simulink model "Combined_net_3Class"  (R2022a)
settings: Solver=FixedStepAuto  StartTime=0.0  StopTime=simtime  FixedStep=1  RelTol=1e-3
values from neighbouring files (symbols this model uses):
  simtime = length(SOC_CC{1, 1})    [Data_preparation.m]    (also in SimulationCycle.m = cell2mat(simtime_og(i)))
  SOH_predict = double(ans.SOHout(simtime))    [SimulationCycle.m]
undefined symbols (not defined in the file or in its folder): dSOC_mu_CC, dSOC_sig_CC, dv_mu_CC, dv_sig_CC, SOC_mu_CC, SOC_sig_CC, SOE_mu_CC, SOE_sig_CC
libraries: neural x121, deeplib x1
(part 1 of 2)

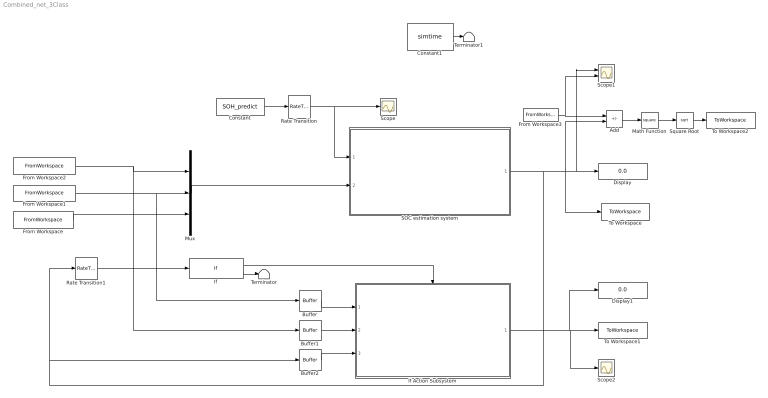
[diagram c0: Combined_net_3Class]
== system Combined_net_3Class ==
  Add : Sum  Inputs=+-
  Buffer : Buffer  N=120  OutputFrames=off
  Buffer1 : Buffer  N=120  OutputFrames=off
  Buffer2 : Buffer  N=120  OutputFrames=off
  Constant : Constant  Value=SOH_predict
  Constant1 : Constant  Value=simtime
  Display : Display
  Display1 : Display
  From Workspace : FromWorkspace  VariableName=Temperature
  From Workspace1 : FromWorkspace  VariableName=Voltage  SampleTime=1
  From Workspace2 : FromWorkspace  VariableName=Current  SampleTime=1
  From Workspace3 : FromWorkspace  VariableName=SOC_GT
  If : If  IfExpression=u1 < 0.6
  If Action Subsystem : Subsystem  TreatAsAtomicUnit=on
  Math Function : Math  Operator=square
  Mux : Mux  Inputs=3
  Rate Transition : RateTransition  OutPortSampleTime=1
  Rate Transition1 : RateTransition  OutPortSampleTime=1
  SOC estimation system : Subsystem
  Scope : Scope
  Scope1 : Scope  NumInputPorts=2
  Scope2 : Scope
  Square Root : Sqrt
  Terminator : Terminator
  Terminator1 : Terminator
  To Workspace : ToWorkspace  VariableName=SOCout  SampleTime=-1
  To Workspace1 : ToWorkspace  VariableName=SOHout  SampleTime=-1
  To Workspace2 : ToWorkspace  VariableName=SOC_abserror  SampleTime=-1
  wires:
  From Workspace/1 -> Mux/3
  Mux/1 -> SOC estimation system/2(Input data)
  If/1 -> If Action Subsystem/Action
  If/2 -> Terminator/1
  Rate Transition1/1 -> If/1
  Buffer2/1 -> If Action Subsystem/3(SOC)
  Buffer1/1 -> If Action Subsystem/2(I)
  From Workspace1/1 -> Buffer/1, Mux/2
  Buffer/1 -> If Action Subsystem/1(V)
  SOC estimation system/1(SOC) -> Scope1/1, Display/1, Add/2, To Workspace/1, Buffer2/1, Rate Transition1/1
  From Workspace2/1 -> Mux/1, Buffer1/1
  If Action Subsystem/1(SOH) -> Display1/1, Scope2/1, To Workspace1/1
  Add/1 -> Math Function/1
  Math Function/1 -> Square Root/1
  Square Root/1 -> To Workspace2/1
  Constant1/1 -> Terminator1/1
  Rate Transition/1 -> SOC estimation system/1(SOH), Scope/1
  From Workspace3/1 -> Add/1, Scope1/2
  Constant/1 -> Rate Transition/1

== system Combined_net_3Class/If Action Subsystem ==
  V : Inport
  I : Inport  Port=2
  SOC : Inport  Port=3
  Action Port : ActionPort  ActionPortLabel=if(u1 < 0.7)
  SOH estimation system : Subsystem
  SOH : Outport
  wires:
  V/1 -> SOH estimation system/1(V)
  I/1 -> SOH estimation system/2(I)
  SOC/1 -> SOH estimation system/3(SOC)
  SOH estimation system/1(Input1) -> SOH/1

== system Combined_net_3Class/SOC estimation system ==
  SOH : Inport
  Input data : Inport  Port=2
  Class1 : Subsystem  TreatAsAtomicUnit=on
  Class2 : Subsystem  TreatAsAtomicUnit=on
  Class3 : Subsystem  TreatAsAtomicUnit=on
  If : If  IfExpression=u1 > 0.93  ElseIfExpressions=u1 <= 0.93 & u1>0.9
  Merge : Merge  Inputs=3
  SOC : Outport
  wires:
  Class2/1(Output) -> Merge/2
  If/1 -> Class1/Action
  Merge/1 -> SOC/1
  Class3/1(Output) -> Merge/3
  Class1/1(Output) -> Merge/1
  SOH/1 -> If/1
  Input data/1 -> Class3/1(Input), Class2/1(Input), Class1/1(Input)
  If/2 -> Class2/Action
  If/3 -> Class3/Action

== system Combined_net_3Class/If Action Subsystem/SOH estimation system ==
  V : Inport
  I : Inport  Port=2
  SOC : Inport  Port=3
  Subsystem1 : Subsystem
  Subsystem2 : Subsystem
  Input1 : Outport
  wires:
  Subsystem1/4(SOE) -> Subsystem2/4(SOE)
  Subsystem1/1(dSOC) -> Subsystem2/1(dSOC)
  Subsystem1/2(dv) -> Subsystem2/2(dv)
  Subsystem1/3(SOC) -> Subsystem2/3(SOC)
  Subsystem2/1(Input1) -> Input1/1
  V/1 -> Subsystem1/1(V_03)
  I/1 -> Subsystem1/2(I_03)
  SOC/1 -> Subsystem1/3(SOC_03)

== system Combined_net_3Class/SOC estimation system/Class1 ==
  Input : Inport
  Action Port : ActionPort  ActionPortLabel=if(u1 > 0.93)
  NARX Neural Network : Subsystem  mask{pi_input_1_delayed_1=[0.507169576059850246707583210081793367862701416015625;-0.464363636363636533843646247987635433673858642578125;-0.84734133790737542479831745367846451699733734130859375], ai_layer_2_delayed_1=-0.99999444038800466838523561818874441087245941162109375}
      mask prompts: pi_input_1_delayed_1 "Preprocessed initial input 1 state at timestep 0."; ai_layer_2_delayed_1 "Initial layer 2 state at timestep 0."
      mask help: NARX Neural Network
  Scope : Scope
  Output : Outport
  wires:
  Input/1 -> NARX Neural Network/1(x)
  NARX Neural Network/1(y) -> Scope/1, Output/1

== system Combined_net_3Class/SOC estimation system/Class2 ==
  Input : Inport
  Action Port : ActionPort  ActionPortLabel=elseif(u1 <= 0.93 & u1>0.9)
  Best class2 NARX Neural Network : Subsystem  mask{pi_input_1_delayed_1=[0.5045468798996550763291679686517454683780670166015625;-0.611404153034653230491812792024575173854827880859375;-1.2613636363636360204765196613152511417865753173828125], ai_layer_2_delayed_1=-0.999993347694183132290390858543105423450469970703125}
      mask prompts: pi_input_1_delayed_1 "Preprocessed initial input 1 state at timestep 0."; ai_layer_2_delayed_1 "Initial layer 2 state at timestep 0."
      mask help: NARX Neural Network
  Scope : Scope
  Output : Outport
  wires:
  Input/1 -> Best class2 NARX Neural Network/1(x)
  Best class2 NARX Neural Network/1(y) -> Scope/1, Output/1

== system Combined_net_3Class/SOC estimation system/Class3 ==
  Input : Inport
  Action Port : ActionPort  ActionPortLabel=else
  New Class 3 NARX Neural Network : Subsystem  mask{pi_input_1_delayed_1=[0.515744420666462755065140299848280847072601318359375;-0.590428999869605064532152027823030948638916015625;-0.633404864091559272054610119084827601909637451171875], ai_layer_2_delayed_1=-0.9999915611182650376775882250512950122356414794921875}
      mask prompts: pi_input_1_delayed_1 "Preprocessed initial input 1 state at timestep 0."; ai_layer_2_delayed_1 "Initial layer 2 state at timestep 0."
      mask help: NARX Neural Network
  Scope : Scope
  Output : Outport
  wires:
  Input/1 -> New Class 3 NARX Neural Network/1(x)
  New Class 3 NARX Neural Network/1(y) -> Scope/1, Output/1

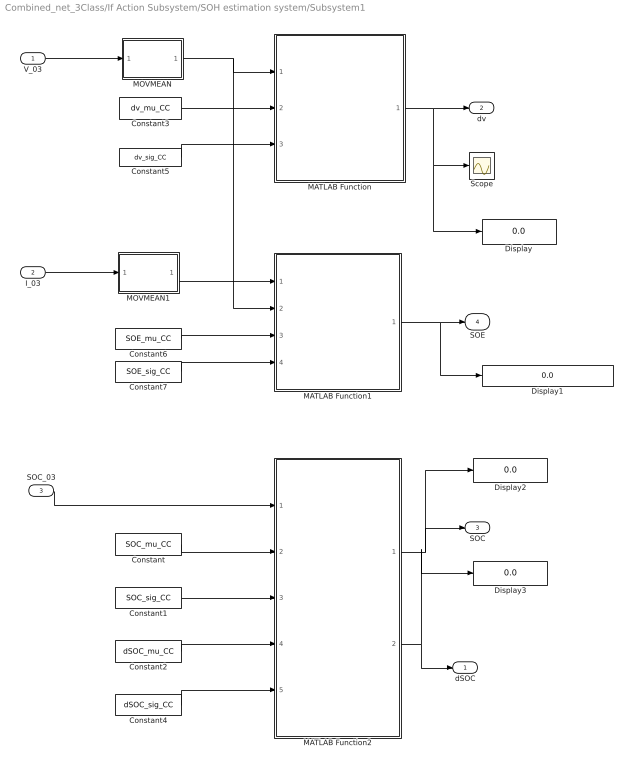
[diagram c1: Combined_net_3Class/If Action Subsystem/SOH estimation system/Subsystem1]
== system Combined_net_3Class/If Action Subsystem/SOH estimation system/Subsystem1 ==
  V_03 : Inport
  I_03 : Inport  Port=2
  SOC_03 : Inport  Port=3
  Constant : Constant  Value=SOC_mu_CC
  Constant1 : Constant  Value=SOC_sig_CC
  Constant2 : Constant  Value=dSOC_mu_CC
  Constant3 : Constant  Value=dv_mu_CC
  Constant4 : Constant  Value=dSOC_sig_CC
  Constant5 : Constant  Value=dv_sig_CC
  Constant6 : Constant  Value=SOE_mu_CC
  Constant7 : Constant  Value=SOE_sig_CC
  Display{,1..3} (4 alike) : Display
  MATLAB Function : MATLAB Function  TreatAsAtomicUnit=on
  MATLAB Function1 : MATLAB Function  TreatAsAtomicUnit=on
  MATLAB Function2 : MATLAB Function  TreatAsAtomicUnit=on
  MOVMEAN : MATLAB Function  TreatAsAtomicUnit=on
  MOVMEAN1 : MATLAB Function  TreatAsAtomicUnit=on
  Scope : Scope
  dSOC : Outport
  dv : Outport  Port=2
  SOC : Outport  Port=3
  SOE : Outport  Port=4
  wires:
  Constant4/1 -> MATLAB Function2/5(dSOC_sig_CC)
  Constant6/1 -> MATLAB Function1/3(SOE_mu_CC)
  Constant7/1 -> MATLAB Function1/4(SOE_sig_CC)
  Constant2/1 -> MATLAB Function2/4(dSOC_mu_CC)
  Constant5/1 -> MATLAB Function/3(dv_sig_CC)
  MATLAB Function2/2(dSOC) -> Display3/1, dSOC/1
  MATLAB Function/1(dV) -> Display/1, Scope/1, dv/1
  MATLAB Function2/1(SOC) -> Display2/1, SOC/1
  Constant3/1 -> MATLAB Function/2(dv_mu_CC)
  V_03/1 -> MOVMEAN/1(V)
  I_03/1 -> MOVMEAN1/1(I)
  Constant1/1 -> MATLAB Function2/3(SOC_sig_CC)
  Constant/1 -> MATLAB Function2/2(SOC_mu_CC)
  MATLAB Function1/1(SOE) -> Display1/1, SOE/1
  MOVMEAN/1(V_filt) -> MATLAB Function/1(V_03), MATLAB Function1/2(V_03)
  MOVMEAN1/1(I_filt) -> MATLAB Function1/1(I_03)
  SOC_03/1 -> MATLAB Function2/1(SOC_03)

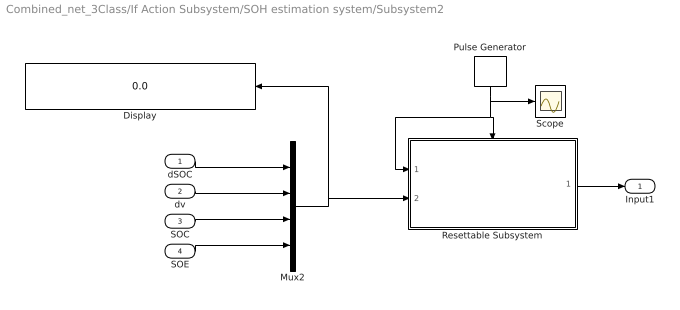
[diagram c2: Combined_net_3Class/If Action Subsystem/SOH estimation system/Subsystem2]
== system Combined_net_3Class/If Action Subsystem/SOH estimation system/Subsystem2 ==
  dSOC : Inport
  dv : Inport  Port=2
  SOC : Inport  Port=3
  SOE : Inport  Port=4
  Display : Display
  Mux2 : Mux
  Pulse Generator : DiscretePulseGenerator  PulseType=Time based  Period=120  PulseWidth=1/120*100  PhaseDelay=119
  Resettable Subsystem : Subsystem  TreatAsAtomicUnit=on
  Scope : Scope
  Input1 : Outport
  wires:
  Mux2/1 -> Display/1, Resettable Subsystem/2(Input1)
  dSOC/1 -> Mux2/1
  dv/1 -> Mux2/2
  SOC/1 -> Mux2/3
  SOE/1 -> Mux2/4
  Pulse Generator/1 -> Resettable Subsystem/1(Input), Resettable Subsystem/Reset, Scope/1
  Resettable Subsystem/1(Out1) -> Input1/1

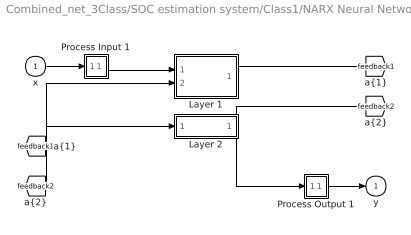
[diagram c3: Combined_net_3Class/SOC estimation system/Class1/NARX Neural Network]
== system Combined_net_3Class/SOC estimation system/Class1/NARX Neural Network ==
  x : Inport  PortDimensions=3  SampleTime=1
  Layer 1 : Subsystem
  Layer 2 : Subsystem
  Process Input 1 : Subsystem
  Process Output 1 : Subsystem
  y : Outport  InitialOutput=0
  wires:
  x/1 -> Process Input 1/1(x)
  Process Output 1/1(y) -> y/1
  Process Input 1/1(p) -> Layer 1/1("p{1}")
  Layer 1/1("a{1}") -> [feedback1]
  [feedback1] -> Layer 2/1("a{1} ")
  Layer 2/1("a{2}") -> [feedback2], Process Output 1/1(a)
  [feedback2] -> Layer 1/2("a{2} ")

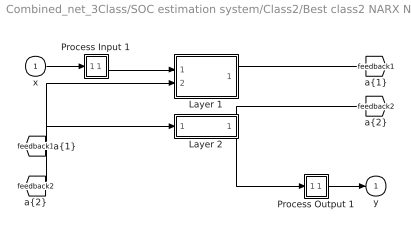
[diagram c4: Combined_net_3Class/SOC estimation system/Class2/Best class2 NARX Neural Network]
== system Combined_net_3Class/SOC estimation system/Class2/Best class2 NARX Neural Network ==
  x : Inport  PortDimensions=3  SampleTime=1
  Layer 1 : Subsystem
  Layer 2 : Subsystem
  Process Input 1 : Subsystem
  Process Output 1 : Subsystem
  y : Outport  InitialOutput=0
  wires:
  x/1 -> Process Input 1/1(x)
  Process Output 1/1(y) -> y/1
  Process Input 1/1(p) -> Layer 1/1("p{1}")
  Layer 1/1("a{1}") -> [feedback1]
  [feedback1] -> Layer 2/1("a{1} ")
  Layer 2/1("a{2}") -> [feedback2], Process Output 1/1(a)
  [feedback2] -> Layer 1/2("a{2} ")

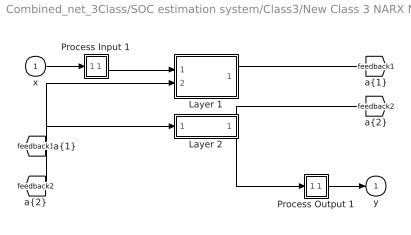
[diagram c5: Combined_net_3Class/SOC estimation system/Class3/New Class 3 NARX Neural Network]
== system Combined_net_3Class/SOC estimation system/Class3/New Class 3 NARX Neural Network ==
  x : Inport  PortDimensions=3  SampleTime=1
  Layer 1 : Subsystem
  Layer 2 : Subsystem
  Process Input 1 : Subsystem
  Process Output 1 : Subsystem
  y : Outport  InitialOutput=0
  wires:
  x/1 -> Process Input 1/1(x)
  Process Output 1/1(y) -> y/1
  Process Input 1/1(p) -> Layer 1/1("p{1}")
  Layer 1/1("a{1}") -> [feedback1]
  [feedback1] -> Layer 2/1("a{1} ")
  Layer 2/1("a{2}") -> [feedback2], Process Output 1/1(a)
  [feedback2] -> Layer 1/2("a{2} ")

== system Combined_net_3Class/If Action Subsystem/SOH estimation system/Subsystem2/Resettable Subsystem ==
  Input : Inport
  Input1 : Inport  Port=2
  Reset : ResetPort  DisableCoverage=on
  Triggered Subsystem : Subsystem  TreatAsAtomicUnit=on
  Out1 : Outport
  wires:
  Triggered Subsystem/1(Out1) -> Out1/1
  Input/1 -> Triggered Subsystem/Trigger
  Input1/1 -> Triggered Subsystem/1(u)

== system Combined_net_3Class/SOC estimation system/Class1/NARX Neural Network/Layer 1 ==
  "p{1}" : Inport  PortDimensions=3  SampleTime=1
  "a{2} " : Inport  Port=2  PortDimensions=1  SampleTime=1
  Delays 1 : Subsystem
  Delays 2 : Subsystem
  "IW{1,1}" : Subsystem
  "LW{1,2}" : Subsystem
  "b{1}" : Constant  Value=[2.272653460716699935773021934437565505504608154296875;1.38176429109038512166307555162347853183746337890625;-1.2278331254825765039839780001784674823284149169921875;-1.605402571388738319768663131981156766414642333984375;-0.32597678534726692856082763682934455573558807373046875;-0.63053100268787576343498813002952374517917633056640625;0.87053292866093390234283333484199829399585723876953125;0.155692044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
  netsum : Sum  Inputs=3  InputSameDT=on  SaturateOnIntegerOverflow=on
  tansig : neural/Transfer Functions/tansig
  "a{1}" : Outport  InitialOutput=[0;0;0;0;0;0;0;0;0;0;0;0;0;0;0;0;0;0;0]
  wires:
  "p{1}"/1 -> Delays 1/1("p{1}")
  Delays 1/1("pd{1,1}") -> "IW{1,1}"/1("pd{1,1}")
  "IW{1,1}"/1("iz{1,1}") -> netsum/1
  "a{2} "/1 -> Delays 2/1("p{1}")
  Delays 2/1("pd{1,2}") -> "LW{1,2}"/1("ad{1,2}")
  "LW{1,2}"/1("lz{1,2}") -> netsum/2
  "b{1}"/1 -> netsum/3
  netsum/1 -> tansig/1
  tansig/1 -> "a{1}"/1

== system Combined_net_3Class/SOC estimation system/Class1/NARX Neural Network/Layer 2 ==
  "a{1} " : Inport  PortDimensions=19  SampleTime=1
  Delays 1 : Subsystem
  "LW{2,1}" : Subsystem
  "b{2}" : Constant  Value=0.1358078901175280017721291869747801683843135833740234375
  netsum : Sum  Inputs=2  InputSameDT=on  SaturateOnIntegerOverflow=on
  purelin : neural/Transfer Functions/purelin
  "a{2}" : Outport  InitialOutput=0
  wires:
  "a{1} "/1 -> Delays 1/1("p{2}")
  Delays 1/1("pd{2,1}") -> "LW{2,1}"/1("ad{2,1}")
  "LW{2,1}"/1("lz{2,1}") -> netsum/1
  "b{2}"/1 -> netsum/2
  netsum/1 -> purelin/1
  purelin/1 -> "a{2}"/1

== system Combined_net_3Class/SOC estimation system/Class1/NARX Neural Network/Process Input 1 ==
  x : Inport  PortDimensions=3  SampleTime=1
  mapminmax : neural/Processing Functions/mapminmax  xmin=[-4.82500000000000017763568394003;2.50609999999999999431565811392;17.9379999999999988347099133534]  xmax=[1.5909999999999999698019337302;4.15610000000000034958702599397;34.2620000000000004547473508865]  ymin=-1  ymax=1
  p : Outport  PortDimensions=3  SampleTime=1
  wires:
  x/1 -> mapminmax/1
  mapminmax/1 -> p/1

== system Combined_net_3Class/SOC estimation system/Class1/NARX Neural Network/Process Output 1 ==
  a : Inport  PortDimensions=1  SampleTime=1
  mapminmax_reverse : neural/Processing Functions/mapminmax_reverse  xmin=-2.77982597386409656609138757455e-06  xmax=1.00000440635255594123975697585  ymin=-1  ymax=1
  y : Outport  PortDimensions=1  SampleTime=1
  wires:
  a/1 -> mapminmax_reverse/1
  mapminmax_reverse/1 -> y/1

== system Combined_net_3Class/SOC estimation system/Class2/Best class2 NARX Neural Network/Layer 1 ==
  "p{1}" : Inport  PortDimensions=3  SampleTime=1
  "a{2} " : Inport  Port=2  PortDimensions=1  SampleTime=1
  Delays 1 : Subsystem
  Delays 2 : Subsystem
  "IW{1,1}" : Subsystem
  "LW{1,2}" : Subsystem
  "b{1}" : Constant  Value=[2.32536033197951841344774948083795607089996337890625;1.6088426828114605893205180109362117946147918701171875;1.839289132479468680259060420212335884571075439453125;1.1409513281229022307883269604644738137722015380859375;-0.84272780046289941235926335139083676040172576904296875;0.8169616653562676855671043085749261081218719482421875;0.8137484932039795726410602583200670778751373291015625;-0.243541688874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
  netsum : Sum  Inputs=3  InputSameDT=on  SaturateOnIntegerOverflow=on
  tansig : neural/Transfer Functions/tansig
  "a{1}" : Outport  InitialOutput=[0;0;0;0;0;0;0;0;0;0;0;0;0;0;0;0;0;0]
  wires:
  "p{1}"/1 -> Delays 1/1("p{1}")
  Delays 1/1("pd{1,1}") -> "IW{1,1}"/1("pd{1,1}")
  "IW{1,1}"/1("iz{1,1}") -> netsum/1
  "a{2} "/1 -> Delays 2/1("p{1}")
  Delays 2/1("pd{1,2}") -> "LW{1,2}"/1("ad{1,2}")
  "LW{1,2}"/1("lz{1,2}") -> netsum/2
  "b{1}"/1 -> netsum/3
  netsum/1 -> tansig/1
  tansig/1 -> "a{1}"/1

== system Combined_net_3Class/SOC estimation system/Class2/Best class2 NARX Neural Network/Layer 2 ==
  "a{1} " : Inport  PortDimensions=18  SampleTime=1
  Delays 1 : Subsystem
  "LW{2,1}" : Subsystem
  "b{2}" : Constant  Value=-0.271815478434470125801425410827505402266979217529296875
  netsum : Sum  Inputs=2  InputSameDT=on  SaturateOnIntegerOverflow=on
  purelin : neural/Transfer Functions/purelin
  "a{2}" : Outport  InitialOutput=0
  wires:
  "a{1} "/1 -> Delays 1/1("p{2}")
  Delays 1/1("pd{2,1}") -> "LW{2,1}"/1("ad{2,1}")
  "LW{2,1}"/1("lz{2,1}") -> netsum/1
  "b{2}"/1 -> netsum/2
  netsum/1 -> purelin/1
  purelin/1 -> "a{2}"/1

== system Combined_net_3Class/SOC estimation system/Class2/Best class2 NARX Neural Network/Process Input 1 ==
  x : Inport  PortDimensions=3  SampleTime=1
  mapminmax : neural/Processing Functions/mapminmax  xmin=[-4.78800000000000025579538487364;2.6570000000000000284217094304;20.6099999999999994315658113919]  xmax=[1.59000000000000007993605777301;4.15470000000000005968558980385;31.5220000000000020179413695587]  ymin=-1  ymax=1
  p : Outport  PortDimensions=3  SampleTime=1
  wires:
  x/1 -> mapminmax/1
  mapminmax/1 -> p/1

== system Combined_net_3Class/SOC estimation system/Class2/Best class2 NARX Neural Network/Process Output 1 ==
  a : Inport  PortDimensions=1  SampleTime=1
  mapminmax_reverse : neural/Processing Functions/mapminmax_reverse  xmin=-3.32617917940104848405083806662e-06  xmax=1.00000457212472371182343522378  ymin=-1  ymax=1
  y : Outport  PortDimensions=1  SampleTime=1
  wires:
  a/1 -> mapminmax_reverse/1
  mapminmax_reverse/1 -> y/1

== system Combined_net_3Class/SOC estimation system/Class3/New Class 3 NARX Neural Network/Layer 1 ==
  "p{1}" : Inport  PortDimensions=3  SampleTime=1
  "a{2} " : Inport  Port=2  PortDimensions=1  SampleTime=1
  Delays 1 : Subsystem
  Delays 2 : Subsystem
  "IW{1,1}" : Subsystem
  "LW{1,2}" : Subsystem
  "b{1}" : Constant  Value=[-2.7411945786634586141872205189429223537445068359375;1.3641694484885682481234425722504965960979461669921875;1.4568466145375698062025549006648361682891845703125;-1.1275543694259562155224330126657150685787200927734375;-0.011340679704705196317870985467379796318709850311279296875;0.2077665605003333748612703857361339032649993896484375;-0.45056896820437841721940230854670517146587371826171875;0.22876919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
  netsum : Sum  Inputs=3  InputSameDT=on  SaturateOnIntegerOverflow=on
  tansig : neural/Transfer Functions/tansig
  "a{1}" : Outport  InitialOutput=[0;0;0;0;0;0;0;0;0;0;0;0;0;0;0;0]
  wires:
  "p{1}"/1 -> Delays 1/1("p{1}")
  Delays 1/1("pd{1,1}") -> "IW{1,1}"/1("pd{1,1}")
  "IW{1,1}"/1("iz{1,1}") -> netsum/1
  "a{2} "/1 -> Delays 2/1("p{1}")
  Delays 2/1("pd{1,2}") -> "LW{1,2}"/1("ad{1,2}")
  "LW{1,2}"/1("lz{1,2}") -> netsum/2
  "b{1}"/1 -> netsum/3
  netsum/1 -> tansig/1
  tansig/1 -> "a{1}"/1

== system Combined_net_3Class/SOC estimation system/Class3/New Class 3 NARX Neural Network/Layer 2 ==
  "a{1} " : Inport  PortDimensions=16  SampleTime=1
  Delays 1 : Subsystem
  "LW{2,1}" : Subsystem
  "b{2}" : Constant  Value=-0.2718737426720261307622195090516470372676849365234375
  netsum : Sum  Inputs=2  InputSameDT=on  SaturateOnIntegerOverflow=on
  purelin : neural/Transfer Functions/purelin
  "a{2}" : Outport  InitialOutput=0
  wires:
  "a{1} "/1 -> Delays 1/1("p{2}")
  Delays 1/1("pd{2,1}") -> "LW{2,1}"/1("ad{2,1}")
  "LW{2,1}"/1("lz{2,1}") -> netsum/1
  "b{2}"/1 -> netsum/2
  netsum/1 -> purelin/1
  purelin/1 -> "a{2}"/1

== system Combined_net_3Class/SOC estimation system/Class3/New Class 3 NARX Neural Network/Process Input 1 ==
  x : Inport  PortDimensions=3  SampleTime=1
  mapminmax : neural/Processing Functions/mapminmax  xmin=[-4.94800000000000039790393202566;2.6339000000000001300293206441;17.1340000000000003410605131648]  xmax=[1.59400000000000008348877145181;4.16769999999999996020960679743;28.3180000000000013926637620898]  ymin=-1  ymax=1
  p : Outport  PortDimensions=3  SampleTime=1
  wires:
  x/1 -> mapminmax/1
  mapminmax/1 -> p/1

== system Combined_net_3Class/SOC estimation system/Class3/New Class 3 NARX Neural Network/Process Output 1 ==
  a : Inport  PortDimensions=1  SampleTime=1
  mapminmax_reverse : neural/Processing Functions/mapminmax_reverse  xmin=-4.21949321457851519659313158095e-06  xmax=1.0000081866738852465203990505  ymin=-1  ymax=1
  y : Outport  PortDimensions=1  SampleTime=1
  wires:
  a/1 -> mapminmax_reverse/1
  mapminmax_reverse/1 -> y/1

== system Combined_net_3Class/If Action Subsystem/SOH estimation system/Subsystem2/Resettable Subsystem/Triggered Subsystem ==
  u : Inport
  Trigger : TriggerPort  TriggerType=falling  VariantControl=(inherit)
  Display : Display
  Scope : Scope
  Stateful Predict : deeplib/Stateful Predict  Network=Network from MAT-file  NetworkFunction=untitled  NetworkFilePath=E:\Thesis\Conclusion step\net.mat  InputDataFormats={ '', '' }  SampleTime=-1  ForceInterpretedSim=off  EnableDLNetwork=on
  Out1 : Outport
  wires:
  u/1 -> Stateful Predict/1, Scope/1, Display/1
  Stateful Predict/1 -> Out1/1

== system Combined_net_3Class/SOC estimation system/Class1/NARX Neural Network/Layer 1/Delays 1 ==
  "p{1}" : Inport  PortDimensions=3  SampleTime=1
  Delay 1 : UnitDelay  InitialCondition=pi_input_1_delayed_1
  mux : Mux  Inputs=2
  "pd{1,1}" : Outport
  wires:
  "p{1}"/1 -> Delay 1/1, mux/1
  Delay 1/1 -> mux/2
  mux/1 -> "pd{1,1}"/1

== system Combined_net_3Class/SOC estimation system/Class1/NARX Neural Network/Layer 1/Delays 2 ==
  "p{1}" : Inport  PortDimensions=1  SampleTime=1
  Delay 1 : UnitDelay  InitialCondition=ai_layer_2_delayed_1
  mux : Mux  Inputs=1
  "pd{1,2}" : Outport
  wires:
  "p{1}"/1 -> Delay 1/1
  Delay 1/1 -> mux/1
  mux/1 -> "pd{1,2}"/1

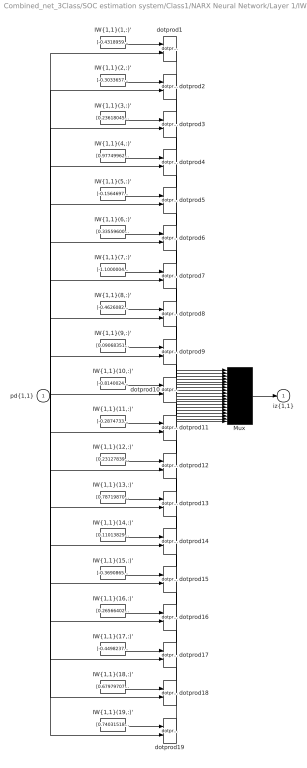
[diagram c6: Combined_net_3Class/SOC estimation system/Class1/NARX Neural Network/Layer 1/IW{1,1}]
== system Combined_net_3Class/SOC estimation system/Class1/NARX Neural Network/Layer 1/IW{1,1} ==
  "pd{1,1}" : Inport  PortDimensions=6  SampleTime=1
  "IW{1,1}(1,:)'" : Constant  Value=[-0.43189597323861317335058629396371543407440185546875;0.73708860161748768202727433163090609014034271240234375;-0.83261969598648211121627582542714662849903106689453125;0.2192268031053078713998871762669296003878116607666015625;1.2068691056179294829320269855088554322719573974609375;1.0400086057173523190755304312915541231632232666015625]
  "IW{1,1}(10,:)'" : Constant  Value=[-0.81400247586885254857946847550920210778713226318359375;0.73570149368374815335158700690953992307186126708984375;-1.1383543127128030736372465980821289122104644775390625;0.77568313249291798161522137888823635876178741455078125;0.56939469605671633178900492566754110157489776611328125;-0.812783732511433765210995261440984904766082763671875]
  "IW{1,1}(11,:)'" : Constant  Value=[-0.287473383298376183869748956567491404712200164794921875;0.2304954461310572966237231185004930011928081512451171875;0.0081437644613669875337524928227139753289520740509033203125;0.2136437142779529507752300787615240551531314849853515625;0.392148852086632526692255851230584084987640380859375;0.1271763362600302205152047463343478739261627197265625]
  "IW{1,1}(12,:)'" : Constant  Value=[0.2312783997838735727814452047823579050600528717041015625;1.203298721703415896655542383086867630481719970703125;0.3695476248105193928239486922393552958965301513671875;-0.61569757708799255357945412470144219696521759033203125;0.801787754423630705247205696650780737400054931640625;0.1214123064778648564132623732803040184080600738525390625]
  "IW{1,1}(13,:)'" : Constant  Value=[0.78719870592613772064538579797954298555850982666015625;-0.62130246056146065658509769491502083837985992431640625;-0.416540846819889731822428302621119655668735504150390625;-0.159244336227894855984033029017155058681964874267578125;-0.464936644334184634441697880902211181819438934326171875;1.0734202509845385264952710713259875774383544921875]
  "IW{1,1}(14,:)'" : Constant  Value=[0.11013829610091063759824692169786430895328521728515625;-0.0935485719430264317519885253204847685992717742919921875;-0.0029358520573019987291718546629226693767122924327850341796875;-0.08321820704705666649214634844611282460391521453857421875;-0.13383849412263248979115815018303692340850830078125;-0.0465056861228394791130114072075230069458484649658203125]
  "IW{1,1}(15,:)'" : Constant  Value=[-0.36908658586228837439335848102928139269351959228515625;0.74551074051353338756342736814985983073711395263671875;1.2712105337784322944827408718992955982685089111328125;0.95631403900313161070556589038460515439510345458984375;-0.76392527146888511424549506045877933502197265625;-0.389063444310004336035291316875373013317584991455078125]
  "IW{1,1}(16,:)'" : Constant  Value=[0.26566402909506958707197554758749902248382568359375;0.2178446778848595055677606069366447627544403076171875;1.29953277841855285856809132383204996585845947265625;0.5980528627707482058895038790069520473480224609375;0.42540531954904892142366179541568271815776824951171875;-0.1626984826696930286349385141875245608389377593994140625]
  "IW{1,1}(17,:)'" : Constant  Value=[-0.4498237183022066876247890832019038498401641845703125;0.3612769768905674805381522673997096717357635498046875;0.01504844182981909632423889178198805893771350383758544921875;0.34152414833792910098253514661337248980998992919921875;0.5469580346102393964002885695663280785083770751953125;0.1833303249193109218939667925951653160154819488525390625]
  "IW{1,1}(18,:)'" : Constant  Value=[0.6797970795831951296150919006322510540485382080078125;-1.1616169096155688489346857750206254422664642333984375;0.0057534012717033004846722832326122443191707134246826171875;-0.5595078694863959700711575351306237280368804931640625;0.1500103731827759079298090227894135750830173492431640625;-0.2156788921534851521943920715784770436584949493408203125]
  "IW{1,1}(19,:)'" : Constant  Value=[0.74031518416065933418934719156823121011257171630859375;0.259378695672205783484542962469276972115039825439453125;-0.1441730104037193538335515086146187968552112579345703125;-0.70054238512878208577916439026012085378170013427734375;0.75000586188900353334929604898206889629364013671875;1.3094986791130571734953491613850928843021392822265625]
  "IW{1,1}(2,:)'" : Constant  Value=[-0.303365708208961415426330177069758065044879913330078125;1.0845316048992279522877879571751691401004791259765625;-0.01744335060242614698911012283133459277451038360595703125;0.319166746750763119511162813068949617445468902587890625;-1.268346430981962758011150071979500353336334228515625;-0.030243487910550030661749332239196519367396831512451171875]
  "IW{1,1}(3,:)'" : Constant  Value=[0.2361804511781558646443812676807283423840999603271484375;-0.1588450949655378641178771204067743383347988128662109375;-0.00878451527350316944964259135986139881424605846405029296875;-0.1775951696259059076066222360168467275798320770263671875;-0.354477096704087391021431585613754577934741973876953125;-0.10745397401892327338135402214902569539844989776611328125]
  "IW{1,1}(4,:)'" : Constant  Value=[0.97749962649128807612441960372962057590484619140625;0.330814652432111555580007689059129916131496429443359375;0.12010836135138154567858492782761459238827228546142578125;-0.96955688937481909750459863062133081257343292236328125;-1.41806698629753835660949334851466119289398193359375;-0.4946472274489597253932515741325914859771728515625]
  "IW{1,1}(5,:)'" : Constant  Value=[-0.1564697266709279277474564651129185222089290618896484375;0.7694512962724540106052018018090166151523590087890625;-0.857499402096217888669116291566751897335052490234375;0.377088498349332945647205406203283928334712982177734375;0.73625718608165258149966803102870471775531768798828125;0.09051525005791115352504760949159390293061733245849609375]
  "IW{1,1}(6,:)'" : Constant  Value=[0.33559600401105071920682121344725601375102996826171875;1.0091141052858392246349694687523879110813140869140625;-0.81312986298143707930563550689839757978916168212890625;0.37091982555840186108753186999820172786712646484375;1.1964018640353726308234172392985783517360687255859375;0.42921359345990184319674654034315608441829681396484375]
  "IW{1,1}(7,:)'" : Constant  Value=[-1.100000423218412404224864076240919530391693115234375;-0.6228561111662986871095881724613718688488006591796875;-0.57604794425345462460796852610656060278415679931640625;0.708887287388822340261640420067124068737030029296875;1.049417107137774252123563201166689395904541015625;-0.928794321351938290121097452356480062007904052734375]
  "IW{1,1}(8,:)'" : Constant  Value=[-0.462608253415409065301133750836015678942203521728515625;0.99003429337342330196491957394755445420742034912109375;1.364558020383528802454975448199547827243804931640625;-0.376520773136293340765945458770147524774074554443359375;0.98233470841508385706930539527093060314655303955078125;0.88107903748410887345698938588611781597137451171875]
  "IW{1,1}(9,:)'" : Constant  Value=[0.090683519999630757268960223882459104061126708984375;0.1462450983808885052184223241056315600872039794921875;0.986033737489041328672101371921598911285400390625;0.1813891768531664394625835257102153263986110687255859375;0.7804879517116611875593434888287447392940521240234375;0.96635327148144012365804655928513966500759124755859375]
  Mux : Mux  Inputs=19
  dotprod{1..19} (19 alike) : neural/Weight Functions/dotprod
  "iz{1,1}" : Outport
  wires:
  "IW{1,1}(1,:)'"/1 -> dotprod1/1
  "pd{1,1}"/1 -> dotprod1/2, dotprod2/2, dotprod3/2, dotprod4/2, dotprod5/2, dotprod6/2, dotprod7/2, dotprod8/2, dotprod9/2, dotprod10/2, dotprod11/2, dotprod12/2, dotprod13/2, dotprod14/2, dotprod15/2, dotprod16/2, dotprod17/2, dotprod18/2, dotprod19/2
  dotprod1/1 -> Mux/1
  "IW{1,1}(2,:)'"/1 -> dotprod2/1
  dotprod2/1 -> Mux/2
  "IW{1,1}(3,:)'"/1 -> dotprod3/1
  dotprod3/1 -> Mux/3
  "IW{1,1}(4,:)'"/1 -> dotprod4/1
  dotprod4/1 -> Mux/4
  "IW{1,1}(5,:)'"/1 -> dotprod5/1
  dotprod5/1 -> Mux/5
  "IW{1,1}(6,:)'"/1 -> dotprod6/1
  dotprod6/1 -> Mux/6
  "IW{1,1}(7,:)'"/1 -> dotprod7/1
  dotprod7/1 -> Mux/7
  "IW{1,1}(8,:)'"/1 -> dotprod8/1
  dotprod8/1 -> Mux/8
  "IW{1,1}(9,:)'"/1 -> dotprod9/1
  dotprod9/1 -> Mux/9
  "IW{1,1}(10,:)'"/1 -> dotprod10/1
  dotprod10/1 -> Mux/10
  "IW{1,1}(11,:)'"/1 -> dotprod11/1
  dotprod11/1 -> Mux/11
  "IW{1,1}(12,:)'"/1 -> dotprod12/1
  dotprod12/1 -> Mux/12
  "IW{1,1}(13,:)'"/1 -> dotprod13/1
  dotprod13/1 -> Mux/13
  "IW{1,1}(14,:)'"/1 -> dotprod14/1
  dotprod14/1 -> Mux/14
  "IW{1,1}(15,:)'"/1 -> dotprod15/1
  dotprod15/1 -> Mux/15
  "IW{1,1}(16,:)'"/1 -> dotprod16/1
  dotprod16/1 -> Mux/16
  "IW{1,1}(17,:)'"/1 -> dotprod17/1
  dotprod17/1 -> Mux/17
  "IW{1,1}(18,:)'"/1 -> dotprod18/1
  dotprod18/1 -> Mux/18
  "IW{1,1}(19,:)'"/1 -> dotprod19/1
  dotprod19/1 -> Mux/19
  Mux/1 -> "iz{1,1}"/1

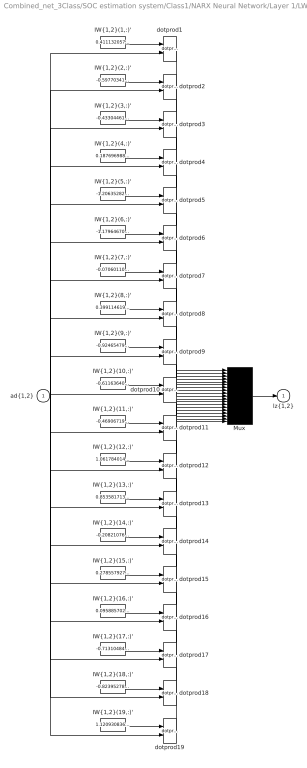
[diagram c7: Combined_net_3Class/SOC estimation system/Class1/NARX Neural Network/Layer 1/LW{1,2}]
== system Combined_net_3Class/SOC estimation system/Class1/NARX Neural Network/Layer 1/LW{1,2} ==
  "ad{1,2}" : Inport  PortDimensions=1  SampleTime=1
  "IW{1,2}(1,:)'" : Constant  Value=0.411132057711244669473416024629841558635234832763671875
  "IW{1,2}(10,:)'" : Constant  Value=-0.61163640576084576938598047490813769400119781494140625
  "IW{1,2}(11,:)'" : Constant  Value=-0.46906719085010550873704460173030383884906768798828125
  "IW{1,2}(12,:)'" : Constant  Value=1.0617840149433048768656817628652788698673248291015625
  "IW{1,2}(13,:)'" : Constant  Value=0.853581713150047161065003820112906396389007568359375
  "IW{1,2}(14,:)'" : Constant  Value=-0.2082107697980564997575214647440589033067226409912109375
  "IW{1,2}(15,:)'" : Constant  Value=0.278557927671726546225983156546135433018207550048828125
  "IW{1,2}(16,:)'" : Constant  Value=0.09588570232729128062221235495599103160202503204345703125
  "IW{1,2}(17,:)'" : Constant  Value=-0.713104840126477679262961828499101102352142333984375
  "IW{1,2}(18,:)'" : Constant  Value=-0.823952784667849602584510648739524185657501220703125
  "IW{1,2}(19,:)'" : Constant  Value=1.1209308364995205220537854984286241233348846435546875
  "IW{1,2}(2,:)'" : Constant  Value=-0.59770341083400280179915853295824490487575531005859375
  "IW{1,2}(3,:)'" : Constant  Value=-0.4330446150937536931024851583060808479785919189453125
  "IW{1,2}(4,:)'" : Constant  Value=0.1876969883577222220072400205026497133076190948486328125
  "IW{1,2}(5,:)'" : Constant  Value=-1.2063528248251864649631670545204542577266693115234375
  "IW{1,2}(6,:)'" : Constant  Value=-1.1796467075375238753309758976683951914310455322265625
  "IW{1,2}(7,:)'" : Constant  Value=-0.07060110044048865940435888433057698421180248260498046875
  "IW{1,2}(8,:)'" : Constant  Value=0.399114619596659447875452997323009185492992401123046875
  "IW{1,2}(9,:)'" : Constant  Value=-0.92465479858880705865686877586995251476764678955078125
  Mux : Mux  Inputs=19
  dotprod{1..19} (19 alike) : neural/Weight Functions/dotprod
  "lz{1,2}" : Outport
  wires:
  "IW{1,2}(1,:)'"/1 -> dotprod1/1
  "ad{1,2}"/1 -> dotprod1/2, dotprod2/2, dotprod3/2, dotprod4/2, dotprod5/2, dotprod6/2, dotprod7/2, dotprod8/2, dotprod9/2, dotprod10/2, dotprod11/2, dotprod12/2, dotprod13/2, dotprod14/2, dotprod15/2, dotprod16/2, dotprod17/2, dotprod18/2, dotprod19/2
  dotprod1/1 -> Mux/1
  "IW{1,2}(2,:)'"/1 -> dotprod2/1
  dotprod2/1 -> Mux/2
  "IW{1,2}(3,:)'"/1 -> dotprod3/1
  dotprod3/1 -> Mux/3
  "IW{1,2}(4,:)'"/1 -> dotprod4/1
  dotprod4/1 -> Mux/4
  "IW{1,2}(5,:)'"/1 -> dotprod5/1
  dotprod5/1 -> Mux/5
  "IW{1,2}(6,:)'"/1 -> dotprod6/1
  dotprod6/1 -> Mux/6
  "IW{1,2}(7,:)'"/1 -> dotprod7/1
  dotprod7/1 -> Mux/7
  "IW{1,2}(8,:)'"/1 -> dotprod8/1
  dotprod8/1 -> Mux/8
  "IW{1,2}(9,:)'"/1 -> dotprod9/1
  dotprod9/1 -> Mux/9
  "IW{1,2}(10,:)'"/1 -> dotprod10/1
  dotprod10/1 -> Mux/10
  "IW{1,2}(11,:)'"/1 -> dotprod11/1
  dotprod11/1 -> Mux/11
  "IW{1,2}(12,:)'"/1 -> dotprod12/1
  dotprod12/1 -> Mux/12
  "IW{1,2}(13,:)'"/1 -> dotprod13/1
  dotprod13/1 -> Mux/13
  "IW{1,2}(14,:)'"/1 -> dotprod14/1
  dotprod14/1 -> Mux/14
  "IW{1,2}(15,:)'"/1 -> dotprod15/1
  dotprod15/1 -> Mux/15
  "IW{1,2}(16,:)'"/1 -> dotprod16/1
  dotprod16/1 -> Mux/16
  "IW{1,2}(17,:)'"/1 -> dotprod17/1
  dotprod17/1 -> Mux/17
  "IW{1,2}(18,:)'"/1 -> dotprod18/1
  dotprod18/1 -> Mux/18
  "IW{1,2}(19,:)'"/1 -> dotprod19/1
  dotprod19/1 -> Mux/19
  Mux/1 -> "lz{1,2}"/1

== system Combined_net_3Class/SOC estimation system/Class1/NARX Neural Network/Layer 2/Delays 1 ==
  "p{2}" : Inport  PortDimensions=19  SampleTime=1
  mux : Mux  Inputs=1
  "pd{2,1}" : Outport
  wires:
  "p{2}"/1 -> mux/1
  mux/1 -> "pd{2,1}"/1

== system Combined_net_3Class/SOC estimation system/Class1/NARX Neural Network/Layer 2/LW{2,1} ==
  "ad{2,1}" : Inport  PortDimensions=19  SampleTime=1
  "IW{2,1}(1,:)'" : Constant  Value=[0.0019784698607019052078725973586870168219320476055145263671875;-0.061192762589771527992343891355631058104336261749267578125;-0.481449370326465564406959174448275007307529449462890625;0.010360444241519654873240341430573607794940471649169921875;-0.0006788650513981395011320341126292987610213458538055419921875;0.000487598912517474562984542973964607881498523056507110595703125;0.00064382068310111053351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
  Mux : Mux  Inputs=1
  dotprod1 : neural/Weight Functions/dotprod
  "lz{2,1}" : Outport
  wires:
  "IW{2,1}(1,:)'"/1 -> dotprod1/1
  "ad{2,1}"/1 -> dotprod1/2
  dotprod1/1 -> Mux/1
  Mux/1 -> "lz{2,1}"/1

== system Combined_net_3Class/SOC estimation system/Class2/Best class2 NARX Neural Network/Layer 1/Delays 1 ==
  "p{1}" : Inport  PortDimensions=3  SampleTime=1
  Delay 1 : UnitDelay  InitialCondition=pi_input_1_delayed_1
  mux : Mux  Inputs=2
  "pd{1,1}" : Outport
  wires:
  "p{1}"/1 -> Delay 1/1, mux/1
  Delay 1/1 -> mux/2
  mux/1 -> "pd{1,1}"/1

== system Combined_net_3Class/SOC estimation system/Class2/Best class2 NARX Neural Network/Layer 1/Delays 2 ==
  "p{1}" : Inport  PortDimensions=1  SampleTime=1
  Delay 1 : UnitDelay  InitialCondition=ai_layer_2_delayed_1
  mux : Mux  Inputs=1
  "pd{1,2}" : Outport
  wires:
  "p{1}"/1 -> Delay 1/1
  Delay 1/1 -> mux/1
  mux/1 -> "pd{1,2}"/1

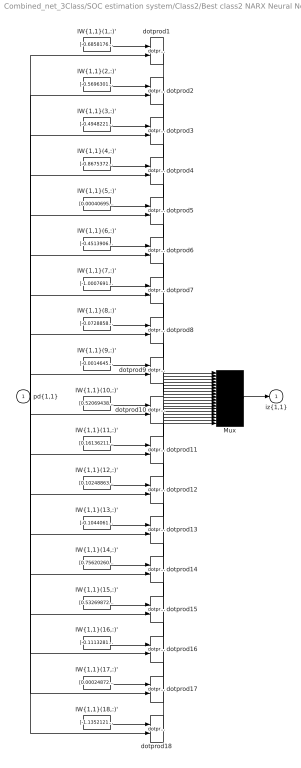
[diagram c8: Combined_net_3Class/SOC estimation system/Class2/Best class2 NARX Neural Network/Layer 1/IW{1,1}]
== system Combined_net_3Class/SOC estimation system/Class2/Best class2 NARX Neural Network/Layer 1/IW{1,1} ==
  "pd{1,1}" : Inport  PortDimensions=6  SampleTime=1
  "IW{1,1}(1,:)'" : Constant  Value=[-0.68581763775791293458183872644440270960330963134765625;-0.456603987743968098289570889392052777111530303955078125;0.958220585278225289727060953737236559391021728515625;-0.331913522723240428380364619442843832075595855712890625;-1.003293923559439360104761362890712916851043701171875;0.550724363129385441339991302811540663242340087890625]
  "IW{1,1}(10,:)'" : Constant  Value=[0.5206943868947140341418844400322996079921722412109375;-0.73737150371318715968982360209338366985321044921875;0.381765347471742177987152899731881916522979736328125;-0.39455145073470754280009487047209404408931732177734375;0.1283544455712402887481715652029379270970821380615234375;-0.25896098034924730502126521969330497086048126220703125]
  "IW{1,1}(11,:)'" : Constant  Value=[0.16136211027004521145755688849021680653095245361328125;-0.448550971866836067913908436821657232940196990966796875;-0.365295790724884827938012676895596086978912353515625;-0.1283731181405824706143192770468886010348796844482421875;-0.08100572907230639552178530493620201013982295989990234375;0.603895755891666663472960863145999610424041748046875]
  "IW{1,1}(12,:)'" : Constant  Value=[0.1024886383532670475204895410570316016674041748046875;0.74539659324562179687490015567163936793804168701171875;0.30591275832944686552394841783097945153713226318359375;-0.071155468095949248041875989656546153128147125244140625;-0.71979006418949198486956220222054980695247650146484375;-0.379590548367549185382330279026064090430736541748046875]
  "IW{1,1}(13,:)'" : Constant  Value=[-0.1044061093258395189753429121992667205631732940673828125;-0.357722011047249932591540755311143584549427032470703125;-0.5986831999460136000124066413263790309429168701171875;-0.70389870950916322289714344151434488594532012939453125;-1.2829672747675908706099789924337528645992279052734375;1.1341694336552234911863479283056221902370452880859375]
  "IW{1,1}(14,:)'" : Constant  Value=[0.75620260636607350424043261227780021727085113525390625;1.26562411313230871456880777259357273578643798828125;-0.03804191663271803969248452403917326591908931732177734375;-0.9124606303781603866553950865636579692363739013671875;-0.04548106944269585116824572423865902237594127655029296875;-0.81484205322189062759008493230794556438922882080078125]
  "IW{1,1}(15,:)'" : Constant  Value=[0.53269872459581002477335687217419035732746124267578125;-0.4747350288887550728844644254422746598720550537109375;-0.56369520990547938854575704681337811052799224853515625;-1.041609846280703077781026877346448600292205810546875;0.382993458021068933216923824147670529782772064208984375;-1.130176476816302066907837797771207988262176513671875]
  "IW{1,1}(16,:)'" : Constant  Value=[-0.11132812564588558112976812708438956178724765777587890625;0.92768503929130685659032451439998112618923187255859375;-0.53849289916432951930147510211099870502948760986328125;-0.0308207664427507278814832858415684313513338565826416015625;-0.52425890354320692221534727650578133761882781982421875;0.577933522035116720161340708727948367595672607421875]
  "IW{1,1}(17,:)'" : Constant  Value=[0.0002487218678451249523515820261110320643638260662555694580078125;0.2106698813322414320925446418186766095459461212158203125;-0.61145243235666324466137666604481637477874755859375;-0.0434297860928491985532673425041139125823974609375;0.97735537938457139883752233799896202981472015380859375;0.10640202899542906822549781509223976172506809234619140625]
  "IW{1,1}(18,:)'" : Constant  Value=[-1.1352121420059944068015056473086588084697723388671875;0.355820212479250830295285368265467695891857147216796875;-0.7534273223966454491318245345610193908214569091796875;-1.0613156657540780969384286436252295970916748046875;-0.43408312608735766247036735876463353633880615234375;-0.54028368641492097168566033360548317432403564453125]
  "IW{1,1}(2,:)'" : Constant  Value=[-0.56963018716061364354885654393001459538936614990234375;-0.7215832884245301226400215455214492976665496826171875;0.76068006441034541342816055475850589573383331298828125;-0.6597900095933566522177216029376722872257232666015625;-0.67896585396289899083654972855583764612674713134765625;0.07665987415377999159016297880953061394393444061279296875]
  "IW{1,1}(3,:)'" : Constant  Value=[-0.49482212198853137152809722465462982654571533203125;0.1342811085264103976300020804046653211116790771484375;0.121182860294636152165281828274601139128208160400390625;-0.03907024287179672317193990238592959940433502197265625;1.387288203272537767674066344625316560268402099609375;-0.92182466643628202529470172521541826426982879638671875]
  "IW{1,1}(4,:)'" : Constant  Value=[-0.8675372373443812623605708722607232630252838134765625;-0.63395237060577980248154972287011332809925079345703125;-0.188537234563857847291501457220874726772308349609375;-1.3949464901580779230272355562192387878894805908203125;-1.0844638394603085540524034513509832322597503662109375;-0.5302770341292895039941868162713944911956787109375]
  "IW{1,1}(5,:)'" : Constant  Value=[0.0004069581202841635590196356364600660526775754988193511962890625;-0.020195033559918730559079591557747335173189640045166015625;0.006676009899000427162685245008333367877639830112457275390625;0.0015061008192939133280841002004990514251403510570526123046875;0.015017663460699361144268237922005937434732913970947265625;-0.00731453578047028089847980680815453524701297283172607421875]
  "IW{1,1}(6,:)'" : Constant  Value=[-0.451390642196218772053128986954106949269771575927734375;-0.75732567538895467773585323811857961118221282958984375;-1.1146372861169180357165942041319794952869415283203125;0.99840100761560501840818915297859348356723785400390625;-0.65859976987469870390867754395003430545330047607421875;-0.73045412029283596222484220561455003917217254638671875]
  "IW{1,1}(7,:)'" : Constant  Value=[-1.000769138545876568713310916791670024394989013671875;-0.76612669930910204385554607142694294452667236328125;-0.84250616646919296304218960358412005007266998291015625;-0.756937399340295247185395055566914379596710205078125;-0.8011577006665564493204101381707005202770233154296875;-0.340688795913904940437788582130451686680316925048828125]
  "IW{1,1}(8,:)'" : Constant  Value=[-0.0728858340014564287656639862689189612865447998046875;0.0719905015437125317401267921013641171157360076904296875;-0.312327053162832879440458100361865945160388946533203125;-0.004339260546920638283996396467045997269451618194580078125;0.136632819861911725123349015120766125619411468505859375;0.34013373875973418325457942046341486275196075439453125]
  "IW{1,1}(9,:)'" : Constant  Value=[-0.0014645233429201550724718661200540736899711191654205322265625;-0.0157623126579764238908154538876260630786418914794921875;-0.004697552812237478468693208100148694938980042934417724609375;0.0012303301726650831514342510075721293105743825435638427734375;0.0136363067416322147895613170476281084120273590087890625;0.006217527091604792797985279406702829874120652675628662109375]
  Mux : Mux  Inputs=18
  dotprod{1..18} (18 alike) : neural/Weight Functions/dotprod
  "iz{1,1}" : Outport
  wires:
  "IW{1,1}(1,:)'"/1 -> dotprod1/1
  "pd{1,1}"/1 -> dotprod1/2, dotprod2/2, dotprod3/2, dotprod4/2, dotprod5/2, dotprod6/2, dotprod7/2, dotprod8/2, dotprod9/2, dotprod10/2, dotprod11/2, dotprod12/2, dotprod13/2, dotprod14/2, dotprod15/2, dotprod16/2, dotprod17/2, dotprod18/2
  dotprod1/1 -> Mux/1
  "IW{1,1}(2,:)'"/1 -> dotprod2/1
  dotprod2/1 -> Mux/2
  "IW{1,1}(3,:)'"/1 -> dotprod3/1
  dotprod3/1 -> Mux/3
  "IW{1,1}(4,:)'"/1 -> dotprod4/1
  dotprod4/1 -> Mux/4
  "IW{1,1}(5,:)'"/1 -> dotprod5/1
  dotprod5/1 -> Mux/5
  "IW{1,1}(6,:)'"/1 -> dotprod6/1
  dotprod6/1 -> Mux/6
  "IW{1,1}(7,:)'"/1 -> dotprod7/1
  dotprod7/1 -> Mux/7
  "IW{1,1}(8,:)'"/1 -> dotprod8/1
  dotprod8/1 -> Mux/8
  "IW{1,1}(9,:)'"/1 -> dotprod9/1
  dotprod9/1 -> Mux/9
  "IW{1,1}(10,:)'"/1 -> dotprod10/1
  dotprod10/1 -> Mux/10
  "IW{1,1}(11,:)'"/1 -> dotprod11/1
  dotprod11/1 -> Mux/11
  "IW{1,1}(12,:)'"/1 -> dotprod12/1
  dotprod12/1 -> Mux/12
  "IW{1,1}(13,:)'"/1 -> dotprod13/1
  dotprod13/1 -> Mux/13
  "IW{1,1}(14,:)'"/1 -> dotprod14/1
  dotprod14/1 -> Mux/14
  "IW{1,1}(15,:)'"/1 -> dotprod15/1
  dotprod15/1 -> Mux/15
  "IW{1,1}(16,:)'"/1 -> dotprod16/1
  dotprod16/1 -> Mux/16
  "IW{1,1}(17,:)'"/1 -> dotprod17/1
  dotprod17/1 -> Mux/17
  "IW{1,1}(18,:)'"/1 -> dotprod18/1
  dotprod18/1 -> Mux/18
  Mux/1 -> "iz{1,1}"/1

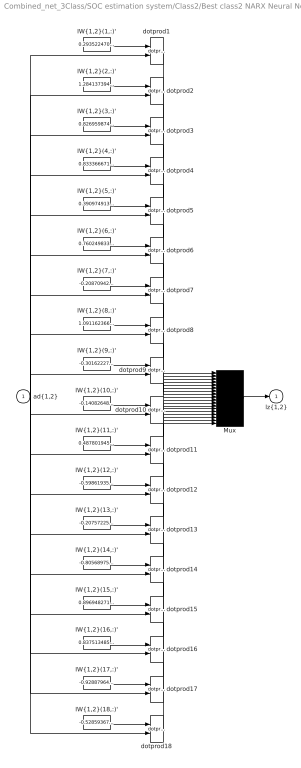
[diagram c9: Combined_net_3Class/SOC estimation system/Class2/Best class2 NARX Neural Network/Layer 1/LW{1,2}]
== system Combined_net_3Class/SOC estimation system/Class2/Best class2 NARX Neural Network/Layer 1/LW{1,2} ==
  "ad{1,2}" : Inport  PortDimensions=1  SampleTime=1
  "IW{1,2}(1,:)'" : Constant  Value=0.2935224701681644621231725977850146591663360595703125
  "IW{1,2}(10,:)'" : Constant  Value=-0.1408264883799905664574225738761015236377716064453125
  "IW{1,2}(11,:)'" : Constant  Value=0.48780194551369293609610622297623194754123687744140625
  "IW{1,2}(12,:)'" : Constant  Value=-0.59861935870906768375476758592412807047367095947265625
  "IW{1,2}(13,:)'" : Constant  Value=-0.207572252376580446142639857498579658567905426025390625
  "IW{1,2}(14,:)'" : Constant  Value=-0.80568975134083309352917012802208773791790008544921875
  "IW{1,2}(15,:)'" : Constant  Value=0.89694827161947154881005417337291873991489410400390625
  "IW{1,2}(16,:)'" : Constant  Value=0.837513485109309119280851518851704895496368408203125
  "IW{1,2}(17,:)'" : Constant  Value=-0.92887964032345615716934617012157104909420013427734375
  "IW{1,2}(18,:)'" : Constant  Value=-0.528593677145003493222930046613328158855438232421875
  "IW{1,2}(2,:)'" : Constant  Value=1.28413739420467987173424262437038123607635498046875
  "IW{1,2}(3,:)'" : Constant  Value=0.82695987492306166632971553553943522274494171142578125
  "IW{1,2}(4,:)'" : Constant  Value=0.83336667184449242373744937140145339071750640869140625
  "IW{1,2}(5,:)'" : Constant  Value=0.3909749131936817168053721616161055862903594970703125
  "IW{1,2}(6,:)'" : Constant  Value=0.76024983306296423091197311805444769561290740966796875
  "IW{1,2}(7,:)'" : Constant  Value=-0.2087094292522974348091935326010570861399173736572265625
  "IW{1,2}(8,:)'" : Constant  Value=1.0911623668276408949395772651769220829010009765625
  "IW{1,2}(9,:)'" : Constant  Value=-0.301622274962787262353458572761155664920806884765625
  Mux : Mux  Inputs=18
  dotprod{1..18} (18 alike) : neural/Weight Functions/dotprod
  "lz{1,2}" : Outport
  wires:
  "IW{1,2}(1,:)'"/1 -> dotprod1/1
  "ad{1,2}"/1 -> dotprod1/2, dotprod2/2, dotprod3/2, dotprod4/2, dotprod5/2, dotprod6/2, dotprod7/2, dotprod8/2, dotprod9/2, dotprod10/2, dotprod11/2, dotprod12/2, dotprod13/2, dotprod14/2, dotprod15/2, dotprod16/2, dotprod17/2, dotprod18/2
  dotprod1/1 -> Mux/1
  "IW{1,2}(2,:)'"/1 -> dotprod2/1
  dotprod2/1 -> Mux/2
  "IW{1,2}(3,:)'"/1 -> dotprod3/1
  dotprod3/1 -> Mux/3
  "IW{1,2}(4,:)'"/1 -> dotprod4/1
  dotprod4/1 -> Mux/4
  "IW{1,2}(5,:)'"/1 -> dotprod5/1
  dotprod5/1 -> Mux/5
  "IW{1,2}(6,:)'"/1 -> dotprod6/1
  dotprod6/1 -> Mux/6
  "IW{1,2}(7,:)'"/1 -> dotprod7/1
  dotprod7/1 -> Mux/7
  "IW{1,2}(8,:)'"/1 -> dotprod8/1
  dotprod8/1 -> Mux/8
  "IW{1,2}(9,:)'"/1 -> dotprod9/1
  dotprod9/1 -> Mux/9
  "IW{1,2}(10,:)'"/1 -> dotprod10/1
  dotprod10/1 -> Mux/10
  "IW{1,2}(11,:)'"/1 -> dotprod11/1
  dotprod11/1 -> Mux/11
  "IW{1,2}(12,:)'"/1 -> dotprod12/1
  dotprod12/1 -> Mux/12
  "IW{1,2}(13,:)'"/1 -> dotprod13/1
  dotprod13/1 -> Mux/13
  "IW{1,2}(14,:)'"/1 -> dotprod14/1
  dotprod14/1 -> Mux/14
  "IW{1,2}(15,:)'"/1 -> dotprod15/1
  dotprod15/1 -> Mux/15
  "IW{1,2}(16,:)'"/1 -> dotprod16/1
  dotprod16/1 -> Mux/16
  "IW{1,2}(17,:)'"/1 -> dotprod17/1
  dotprod17/1 -> Mux/17
  "IW{1,2}(18,:)'"/1 -> dotprod18/1
  dotprod18/1 -> Mux/18
  Mux/1 -> "lz{1,2}"/1

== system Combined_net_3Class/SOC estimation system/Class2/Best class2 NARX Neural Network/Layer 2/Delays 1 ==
  "p{2}" : Inport  PortDimensions=18  SampleTime=1
  mux : Mux  Inputs=1
  "pd{2,1}" : Outport
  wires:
  "p{2}"/1 -> mux/1
  mux/1 -> "pd{2,1}"/1

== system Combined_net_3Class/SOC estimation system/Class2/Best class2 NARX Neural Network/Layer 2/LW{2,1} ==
  "ad{2,1}" : Inport  PortDimensions=18  SampleTime=1
  "IW{2,1}(1,:)'" : Constant  Value=[4.1460602019561805346714589148859886336140334606170654296875e-05;-8.857324199911309806597381477644148617400787770748138427734375e-05;0.0004216897422409032823546748414145213246229104697704315185546875;8.02798038632267381940754713554042609757743775844573974609375e-05;1.7004445865470483312265059794299304485321044921875;-3.043324545280591582742217571233567241506534628570079803466796875e-05;-0.0001508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
  Mux : Mux  Inputs=1
  dotprod1 : neural/Weight Functions/dotprod
  "lz{2,1}" : Outport
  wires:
  "IW{2,1}(1,:)'"/1 -> dotprod1/1
  "ad{2,1}"/1 -> dotprod1/2
  dotprod1/1 -> Mux/1
  Mux/1 -> "lz{2,1}"/1

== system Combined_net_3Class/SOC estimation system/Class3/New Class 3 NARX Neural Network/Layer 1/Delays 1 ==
  "p{1}" : Inport  PortDimensions=3  SampleTime=1
  Delay 1 : UnitDelay  InitialCondition=pi_input_1_delayed_1
  mux : Mux  Inputs=2
  "pd{1,1}" : Outport
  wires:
  "p{1}"/1 -> Delay 1/1, mux/1
  Delay 1/1 -> mux/2
  mux/1 -> "pd{1,1}"/1

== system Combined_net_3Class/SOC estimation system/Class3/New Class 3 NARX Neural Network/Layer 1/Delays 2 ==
  "p{1}" : Inport  PortDimensions=1  SampleTime=1
  Delay 1 : UnitDelay  InitialCondition=ai_layer_2_delayed_1
  mux : Mux  Inputs=1
  "pd{1,2}" : Outport
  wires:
  "p{1}"/1 -> Delay 1/1
  Delay 1/1 -> mux/1
  mux/1 -> "pd{1,2}"/1
